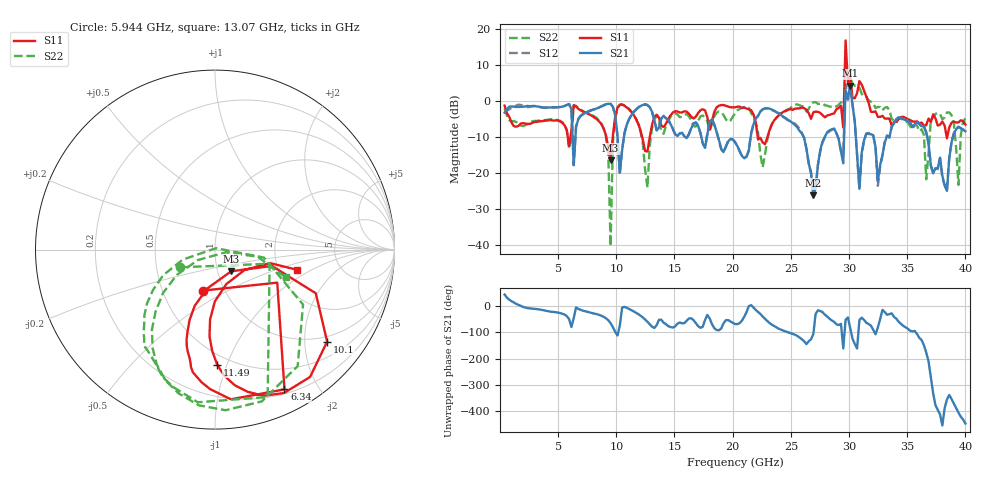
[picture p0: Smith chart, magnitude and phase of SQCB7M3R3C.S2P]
! Network Analyzer HP8722ES.07.66: Jul 25, 2000 Serial No. US39175408
! 26 Oct 2004  13:55:15
! Frequency  S11  S21  S12  S22
# HZ  S  DB R  50
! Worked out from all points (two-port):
!   201 points, 400 MHz to 40 GHz, reference 50 ohm
!   highest |S21| = 4.24 dB at 30.1 GHz (marker M1); lowest = -26.1 dB at 26.93 GHz (marker M2)
!   |S21| within 3 dB of the highest: 29.69 GHz to 29.84 GHz (158 MHz wide, 0.531 % of centre); 29.94 GHz to 30.21 GHz (272.9 MHz wide, 0.907 % of centre)
!   lowest |S11| = -16.4 dB at 9.508 GHz (marker M3), VSWR 1.36, Z = 58 - j14.4 ohm
!   |S11| at or under -10 dB: 9.137 GHz to 9.695 GHz (557.9 MHz wide, 5.92 % of centre); 12.22 GHz to 12.87 GHz (652.7 MHz wide, 5.2 % of centre); 22.15 GHz to 22.99 GHz (837.4 MHz wide, 3.71 % of centre)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
!   |S22| runs from -40.2 to 6.6 dB; largest |S21 - S12| = 0.89
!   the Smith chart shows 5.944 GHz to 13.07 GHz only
!   S11 on the Smith chart (normalised r, x): 5.944 GHz: 0.79, -0.38; 6.34 GHz: 0.25, -1.59; 10.1 GHz: 0.86, -2.54; 11.49 GHz: 0.43, -0.92; 13.07 GHz: 2.52, -0.72
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4e8  -1.29 -48.3  -3.24 43.5  -3.45 48.8  -2.10 -39.7
5.944e9  -12.48 -106.1  -0.86 -50.0  -0.86 -50.6  -13.30 -152.9
6.34e9  -1.21 -63.6  -17.77 -45.9  -17.79 -36.4  -1.19 -70.3
7.132e9  -2.99 -98.8  -3.66 -17.7  -3.71 -18.7  -2.82 -116.7
9.508e9  -16.43 -53.4  -0.84 -65.0  -0.79 -66.1  -40.20 54.3
1.0102e10  -1.85 -39.4  -9.60 -111.9  -9.82 -112.9  -1.98 -54.6
1.1488e10  -3.87 -88.9  -3.09 -20.3  -3.11 -21.0  -3.74 -122.3
1.3072e10  -6.60 -13.8  -2.97 -78.8  -3.09 -79.6  -7.46 -21.5
1.3666e10  -4.65 -46.7  -7.34 -52.4  -7.24 -51.4  -5.42 -68.3
2.02e10  -1.77 -25.1  -11.48 -68.4  -11.30 -67.5  -3.42 -28.7
2.6932e10  -3.15 -119.3  -26.13 -106.3  -25.51 -104.9  -0.38 -2.5
2.9506e10  -7.39 23.5  -17.28 -161.0  -14.48 -108.4  -0.02 26.7
2.9704e10  16.74 -45.3  3.02 -52.3  4.62 -20.6  2.64 -48.5
2.9902e10  4.91 -63.7  0.52 -43.3  0.34 -42.7  4.67 2.3
3.01e10  7.13 -101.9  4.24 -82.8  4.24 -83.4  6.62 -20.1
3.0496e10  0.76 -82.2  -5.79 -144.0  -5.82 -143.3  4.21 -50.2
3.0694e10  2.18 92.7  -14.86 -161.5  -14.89 -158.7  4.12 122.4
3.0892e10  5.48 82.6  -24.34 -53.0  -24.27 -50.6  3.65 114.5
3.1288e10  2.82 18.2  -10.92 -52.7  -10.97 -51.9  1.11 106.8
3.1486e10  1.18 -163.1  -9.00 -63.4  -9.09 -64.1  1.17 -79.0
3.3466e10  -4.89 -168.8  -10.14 -31.0  -10.08 -29.8  -2.52 -125.3
4e10  -6.55 -157.2  -8.39 -86.3  -8.41 -85.1  -4.80 92.6
